(* Logix 5000 DataType export RSG3E_Seneca_InData; software revision 35.00 *)

TYPE RSG3E_Seneca_InData :   // User Define Measure Data Type for Seneca R-SG3-E Device
STRUCT
   DIN1 : BOOL;
   DIN2 : BOOL;
   NET : REAL;
   GROSS : REAL;
   TARE : REAL;
   MAX_NET : REAL;
   MIN_NET : REAL;
   ADC_RAW : UDINT;
   NUM_PIECES : INT;
   STATUS : INT;
END_STRUCT
END_TYPE
